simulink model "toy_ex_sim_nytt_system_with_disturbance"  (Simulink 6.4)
settings: Solver=ode4  StartTime=0.0  StopTime=simtid  FixedStep=.05  RelTol=1e-5
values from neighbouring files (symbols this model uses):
  alpha = -0.9    [bounds.m]    (also in real_ex_linkomb_W_and_DP.m = 1; real_ex_linkomb_W_and_RHOT.m = -0.2; real_ex_without_noise_z_30.m = -6:0.01:4; toy_ex_nytt_system.m)
  den_G1 = [-1 1]    [bounds.m]    (also in toy_ex_nytt_system.m; toy_ex_nytt_system_without_noise.m; toy_ex_nytt_system_with_disturbance.m; toy_ex_nytt_system_with_measure_noise.m)
  den_G2 = [-1 1]    [bounds.m]    (also in toy_ex_nytt_system.m; toy_ex_nytt_system_without_noise.m; toy_ex_nytt_system_with_disturbance.m; toy_ex_nytt_system_with_measure_noise.m)
  K_indre = 10    [real_ex_linkomb_W_and_DP.m]    (also in real_ex_linkomb_W_and_RHOT.m = 5; toy_ex_nytt_system.m = 50; toy_ex_nytt_system_without_noise.m = 20; toy_ex_nytt_system_with_disturbance.m = 50)
  K_ytre = 0.01    [real_ex_linkomb_W_and_DP.m]    (also in real_ex_linkomb_W_and_RHOT.m; toy_ex_nytt_system.m = 0.1; toy_ex_nytt_system_without_noise.m = 0.1; toy_ex_nytt_system_with_disturbance.m = 0.1)
  num_G1 = 5*[-1.5 1]    [bounds.m]    (also in toy_ex_nytt_system.m; toy_ex_nytt_system_without_noise.m; toy_ex_nytt_system_with_disturbance.m; toy_ex_nytt_system_with_measure_noise.m)
  num_G2 = 5*[-0.5 1]    [bounds.m]    (also in toy_ex_nytt_system.m; toy_ex_nytt_system_without_noise.m; toy_ex_nytt_system_with_disturbance.m; toy_ex_nytt_system_with_measure_noise.m)
  Ti = 100    [real_ex_linkomb_W_and_DP.m]    (also in real_ex_linkomb_W_and_RHOT.m = 100000; toy_ex_nytt_system.m = 10; toy_ex_nytt_system_without_noise.m = 10; toy_ex_nytt_system_with_disturbance.m = 10)

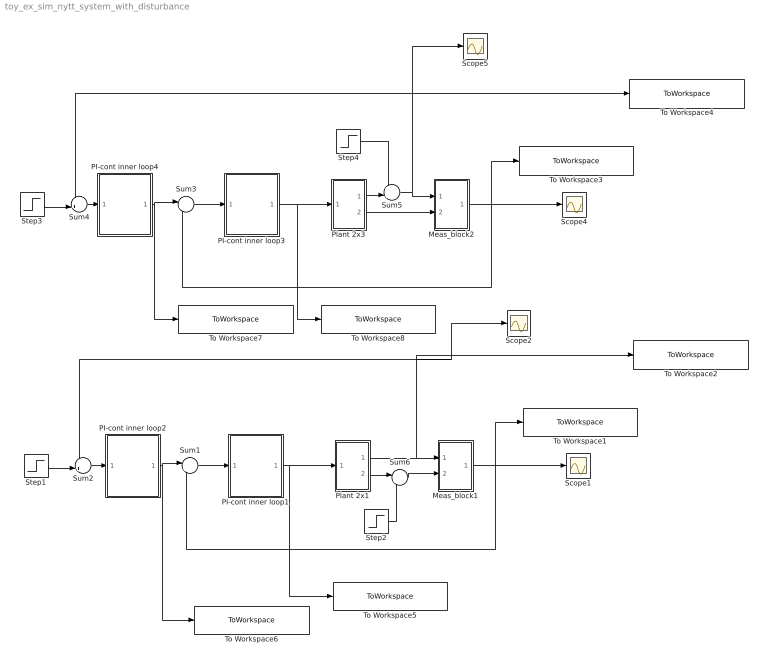
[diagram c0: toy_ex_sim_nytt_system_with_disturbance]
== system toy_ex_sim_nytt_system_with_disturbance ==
  Meas_block1 : Subsystem
  Meas_block2 : Subsystem
  PI-cont inner loop1 : Subsystem
  PI-cont inner loop2 : Subsystem
  PI-cont inner loop3 : Subsystem
  PI-cont inner loop4 : Subsystem
  Plant 2x1 : Subsystem
  Plant 2x3 : Subsystem
  Scope{1..2,4..5} (4 alike) : Scope
  Step1 : Step  Time=0  After=0  SampleTime=0
  Step2 : Step  Time=10  SampleTime=0
  Step3 : Step  Time=0  After=0  SampleTime=0
  Step4 : Step  Time=10  SampleTime=0
  Sum1 : Sum  Inputs=|+-
  Sum2 : Sum  Inputs=-+|
  Sum3 : Sum  Inputs=|+-
  Sum4 : Sum  Inputs=-+|
  Sum5 : Sum  Inputs=++|
  Sum6 : Sum  Inputs=|++
  To Workspace1 : ToWorkspace  VariableName=meas_linkomb2_dist1  SampleTime=-1  SaveFormat=Structure With Time
  To Workspace2 : ToWorkspace  VariableName=meas_y1_dist1  SampleTime=-1  SaveFormat=Structure With Time
  To Workspace3 : ToWorkspace  VariableName=meas_linkomb2_dist  SampleTime=-1  SaveFormat=Structure With Time
  To Workspace4 : ToWorkspace  VariableName=meas_y1_dist  SampleTime=-1  SaveFormat=Structure With Time
  To Workspace5 : ToWorkspace  VariableName=u_inner_disturb_y2  SampleTime=-1  SaveFormat=Structure With Time
  To Workspace6 : ToWorkspace  VariableName=u_outer_disturb_y2  SampleTime=-1  SaveFormat=Structure With Time
  To Workspace7 : ToWorkspace  VariableName=u_outer_disturb_y1  SampleTime=-1  SaveFormat=Structure With Time
  To Workspace8 : ToWorkspace  VariableName=u_inner_disturb_y1  SampleTime=-1  SaveFormat=Structure With Time
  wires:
  Plant 2x3/2(y2) -> Meas_block2/2(In2)
  Meas_block2/1(Out1) -> Sum3/2, Scope4/1, To Workspace3/1
  Sum3/1 -> PI-cont inner loop3/1(In1)
  PI-cont inner loop3/1(Out1) -> Plant 2x3/1(In1), To Workspace8/1
  PI-cont inner loop4/1(Out1) -> Sum3/1, To Workspace7/1
  Step3/1 -> Sum4/2
  Sum4/1 -> PI-cont inner loop4/1(In1)
  Step4/1 -> Sum5/1
  Plant 2x3/1("y1 ") -> Sum5/2
  Sum5/1 -> Meas_block2/1(In1), To Workspace4/1, Scope5/1, Sum4/1
  Meas_block1/1(Out1) -> To Workspace1/1, Scope1/1, Sum1/2
  Sum1/1 -> PI-cont inner loop1/1(In1)
  PI-cont inner loop1/1(Out1) -> Plant 2x1/1(In1), To Workspace5/1
  PI-cont inner loop2/1(Out1) -> Sum1/1, To Workspace6/1
  Step1/1 -> Sum2/2
  Sum2/1 -> PI-cont inner loop2/1(In1)
  Plant 2x1/1("y1 ") -> Sum2/1, Scope2/1, To Workspace2/1, Meas_block1/1(In1)
  Plant 2x1/2(y2) -> Sum6/1
  Sum6/1 -> Meas_block1/2(In2)
  Step2/1 -> Sum6/2

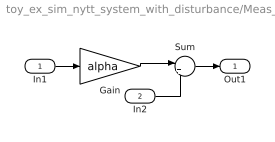
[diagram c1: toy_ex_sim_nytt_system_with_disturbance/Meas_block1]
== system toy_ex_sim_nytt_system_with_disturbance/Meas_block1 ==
  In1 : Inport
  In2 : Inport  Port=2
  Gain : Gain  Gain=alpha
  Sum : Sum  Inputs=|++
  Out1 : Outport
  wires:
  In2/1 -> Sum/2
  Sum/1 -> Out1/1
  In1/1 -> Gain/1
  Gain/1 -> Sum/1

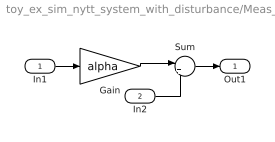
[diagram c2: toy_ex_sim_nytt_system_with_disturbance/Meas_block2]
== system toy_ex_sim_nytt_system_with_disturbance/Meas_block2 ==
  In1 : Inport
  In2 : Inport  Port=2
  Gain : Gain  Gain=alpha
  Sum : Sum  Inputs=|++
  Out1 : Outport
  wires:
  Gain/1 -> Sum/1
  In1/1 -> Gain/1
  Sum/1 -> Out1/1
  In2/1 -> Sum/2

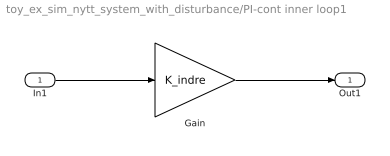
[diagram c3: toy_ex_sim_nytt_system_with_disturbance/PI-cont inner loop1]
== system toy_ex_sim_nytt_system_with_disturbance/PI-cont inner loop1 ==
  In1 : Inport
  Gain : Gain  Gain=K_indre
  Out1 : Outport
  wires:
  In1/1 -> Gain/1
  Gain/1 -> Out1/1

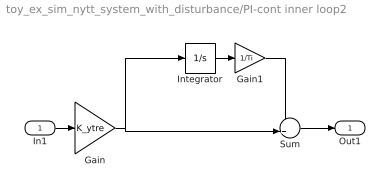
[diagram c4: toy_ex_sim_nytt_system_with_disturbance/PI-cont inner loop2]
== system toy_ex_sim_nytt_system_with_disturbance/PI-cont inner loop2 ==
  In1 : Inport
  Gain : Gain  Gain=K_ytre
  Gain1 : Gain  Gain=1/Ti
  Integrator : Integrator
  Sum : Sum  Inputs=++|
  Out1 : Outport
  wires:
  Gain/1 -> Integrator/1, Sum/2
  In1/1 -> Gain/1
  Integrator/1 -> Gain1/1
  Gain1/1 -> Sum/1
  Sum/1 -> Out1/1

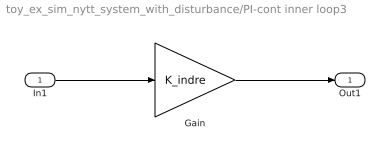
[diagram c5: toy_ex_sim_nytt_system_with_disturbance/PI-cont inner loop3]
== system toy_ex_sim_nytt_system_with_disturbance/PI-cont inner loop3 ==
  In1 : Inport
  Gain : Gain  Gain=K_indre
  Out1 : Outport
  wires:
  Gain/1 -> Out1/1
  In1/1 -> Gain/1

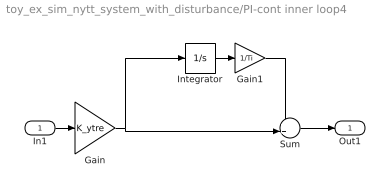
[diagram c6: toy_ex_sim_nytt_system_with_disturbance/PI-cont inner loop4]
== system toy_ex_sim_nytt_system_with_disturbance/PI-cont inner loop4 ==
  In1 : Inport
  Gain : Gain  Gain=K_ytre
  Gain1 : Gain  Gain=1/Ti
  Integrator : Integrator
  Sum : Sum  Inputs=++|
  Out1 : Outport
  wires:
  Sum/1 -> Out1/1
  Gain1/1 -> Sum/1
  Integrator/1 -> Gain1/1
  In1/1 -> Gain/1
  Gain/1 -> Sum/2, Integrator/1

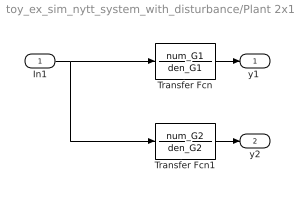
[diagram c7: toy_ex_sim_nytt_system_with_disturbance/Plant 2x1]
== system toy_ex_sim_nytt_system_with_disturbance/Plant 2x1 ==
  In1 : Inport
  Transfer Fcn : TransferFcn  Numerator=num_G1  Denominator=den_G1
  Transfer Fcn1 : TransferFcn  Numerator=num_G2  Denominator=den_G2
  "y1 " : Outport
  y2 : Outport  Port=2
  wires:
  Transfer Fcn1/1 -> y2/1
  Transfer Fcn/1 -> "y1 "/1
  In1/1 -> Transfer Fcn/1, Transfer Fcn1/1

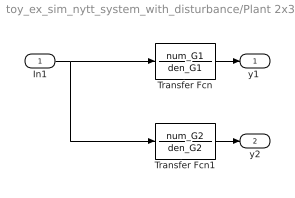
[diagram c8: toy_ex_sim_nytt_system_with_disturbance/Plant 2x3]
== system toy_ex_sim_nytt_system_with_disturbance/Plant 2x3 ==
  In1 : Inport
  Transfer Fcn : TransferFcn  Numerator=num_G1  Denominator=den_G1
  Transfer Fcn1 : TransferFcn  Numerator=num_G2  Denominator=den_G2
  "y1 " : Outport
  y2 : Outport  Port=2
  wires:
  In1/1 -> Transfer Fcn1/1, Transfer Fcn/1
  Transfer Fcn/1 -> "y1 "/1
  Transfer Fcn1/1 -> y2/1
